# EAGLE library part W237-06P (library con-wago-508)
WAGO SREW CLAMP
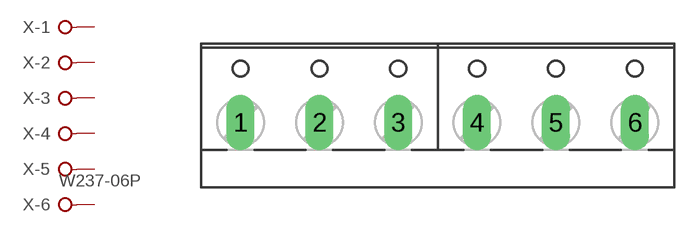
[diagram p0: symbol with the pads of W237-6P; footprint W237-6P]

Designator prefix X; gates -1=KL -2=KL -3=KL -4=KL -5=KL -6=KL+V

## W237-06P (OC_FARNELL: unknown; OC_NEWARK: unknown)  [W237-6P]
1  -1:KL  pas
2  -2:KL  pas
3  -3:KL  pas
4  -4:KL  pas
5  -5:KL  pas
6  -6:KL  pas

## Footprint W237-6P (pad centres in mm)
WAGO SREW CLAMP
drill 1.194 long: 1 -12.7,-0.635; 2 -7.62,-0.635; 3 -2.54,-0.635; 4 2.54,-0.635; 5 7.62,-0.635; 6 12.7,-0.635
